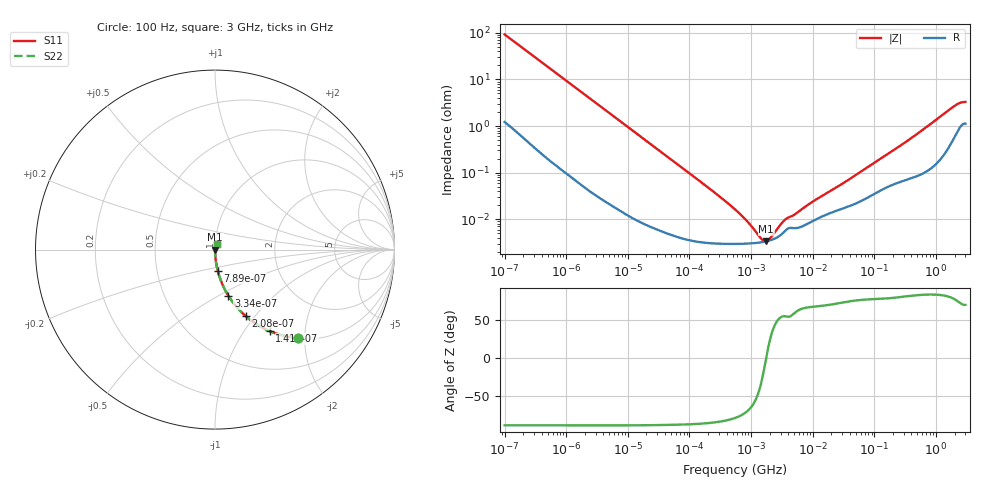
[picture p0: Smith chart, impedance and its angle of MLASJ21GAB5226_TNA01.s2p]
! MLASJ21GAB5226_TNA01  S-PARAMETER MODEL  ( Standard Model )
! Model Generated by TAIYO YUDEN Corporation (http://www.ty-top.com)
! Version 1.0
! TAIYO YUDEN Control No. 220601
! Copyright(c) 2009 TAIYO YUDEN CO.,LTD. All Rights Reserved.
! Product Description (link to TY-COMPAS)
! https://ds.yuden.co.jp/TYCOMPAS/or/detail?pn=MLASJ21GAB5226KTNA01&u=M
! Products Name : Multilayer Ceramic Capacitors
! Characteristics :
!  Capacitance : 22 [uF] , Rated Voltage : 6.3 [V] , TCC : X5R
!  Case Size : 2.0 x 1.25 / 0.079 x 0.049 [mm/inch] , Thickness : 1.25 / 0.049 [mm/inch]
!  (Conditions: Temperature = 25 [degC] , DC Bias Voltage = 0 [V])
! External Node Assignments :
!  1  o---| |---o  2
! GND o---------o GND
! Frequency Range : 100Hz  -  3GHz  [ 401 STEP ]
# MHZ S RI R 50
! Freq[MHz].  S11 Real  S11 Imag  S21 Real  S21 Imag  S12 Real  S12 Imag  S22 Real  S22 Imag
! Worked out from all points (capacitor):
!   401 points, 100 Hz to 3 GHz, reference 50 ohm
!   read as one part in series: C = 17.2 uF near 109 Hz
!   lowest |Z| = 3.34 mohm at 1.751 MHz (marker M1)
!   series resonance near 1.759 MHz, so ESL is about 480 pH
!   S11 on the Smith chart (normalised r, x): 100 Hz: 1.02, -1.85; 141 Hz: 1.02, -1.32; 208 Hz: 1.01, -0.90; 334 Hz: 1.01, -0.56; 789 Hz: 1.00, -0.24; 3 GHz: 1.02, +0.06
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0.0001  0.4617 -0.492  0.5383 0.492  0.5383 0.492  0.4617 -0.492
0.000141  0.3044 -0.4538  0.6956 0.4538  0.6956 0.4538  0.3044 -0.4538
0.000208  0.1702 -0.3699  0.8298 0.3699  0.8298 0.3699  0.1702 -0.3699
0.000334  0.0751 -0.2582  0.9249 0.2582  0.9249 0.2582  0.0751 -0.2582
0.000789  0.0151 -0.1171  0.9849 0.1171  0.9849 0.1171  0.0151 -0.1171
0.001788  0.00331 -0.0526  0.9967 0.0526  0.9967 0.0526  0.00331 -0.0526
0.005476  0.000496 -0.0173  0.9995 0.0173  0.9995 0.0173  0.000496 -0.0173
0.031977  6.66e-05 -0.003  0.9999 0.003  0.9999 0.003  6.66e-05 -0.003
0.221826  3.06e-05 -0.000431  1 0.000431  1 0.000431  3.06e-05 -0.000431
0.547723  2.95e-05 -0.00016  1 0.00016  1 0.00016  2.95e-05 -0.00016
0.740304  2.97e-05 -0.000108  1 0.000108  1 0.000108  2.97e-05 -0.000108
0.842342  2.99e-05 -8.89e-05  1 8.89e-05  1 8.89e-05  2.99e-05 -8.89e-05
1.75092  3.34e-05 -4.93e-07  1 4.93e-07  1 4.93e-07  3.34e-05 -4.93e-07
3.79959  6.05e-05 8.51e-05  0.9999 -8.51e-05  0.9999 -8.51e-05  6.05e-05 8.51e-05
5.135543  6.42e-05 0.00011  0.9999 -0.00011  0.9999 -0.00011  6.42e-05 0.00011
9.794414  8.98e-05 0.000216  0.9999 -0.000216  0.9999 -0.000216  8.98e-05 0.000216
34.12477  0.000178 0.000614  0.9998 -0.000614  0.9998 -0.000614  0.000178 0.000614
175.1444  0.000518 0.0026  0.9995 -0.0026  0.9995 -0.0026  0.000518 0.0026
471.3361  0.000861 0.00641  0.9991 -0.00641  0.9991 -0.00641  0.000861 0.00641
1950.712  0.00609 0.0256  0.9939 -0.0256  0.9939 -0.0256  0.00609 0.0256
2419.119  0.00991 0.0293  0.9901 -0.0293  0.9901 -0.0293  0.00991 0.0293
3000  0.012 0.0303  0.988 -0.0303  0.988 -0.0303  0.012 0.0303
